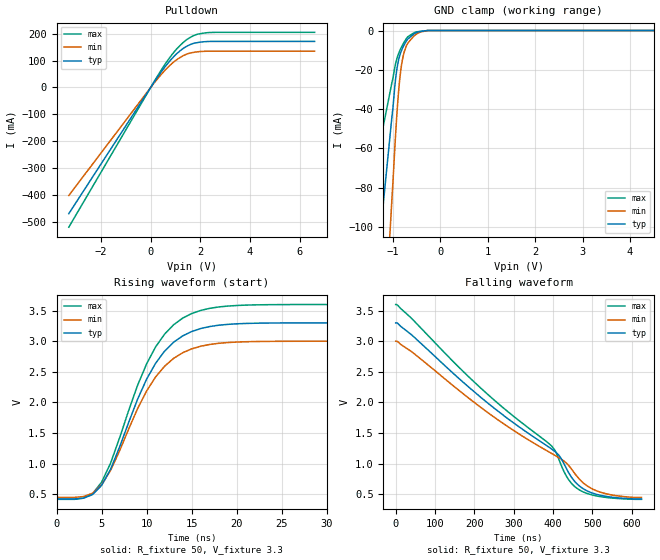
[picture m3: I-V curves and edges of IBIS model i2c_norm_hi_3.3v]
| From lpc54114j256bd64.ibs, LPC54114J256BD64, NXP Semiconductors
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[Model]   i2c_norm_hi_3.3v
Model_type I/O_open_drain
Vinl=8.000E-01
Vinh=2.000E+00
Vref=3.300E+00
Rref=1.000E+03
Cref=0.000E+00
Vmeas=1.650E+00
C_comp   1.270E-12   1.260E-12   1.280E-12
[Voltage Range]   3.300E+00   3.000E+00   3.600E+00
[POWER Clamp Reference]   3.300E+00   3.000E+00   3.600E+00
[GND Clamp Reference]   0.000E+00   0.000E+00   0.000E+00
[Pullup Reference]   3.300E+00   3.000E+00   3.600E+00
[Pulldown Reference]   0.000E+00   0.000E+00   0.000E+00
[Temperature Range]   25   105   -40
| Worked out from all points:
|   slope of the pulldown table from 0 to 0.495 V, typ, clamps not added: 7.43 ohm
|   GND clamp passes 1 mA (typ) near -0.50 V on its own axis
|   rising waveform, R_fixture 50, V_fixture 3.3: 20-80 % time 5.17ns typ, 5.19ns min, 5.15ns max; typ from 0.423 V to 3.3 V
|   falling waveform, R_fixture 50, V_fixture 3.3: 20-80 % time 323ns typ, 336ns min, 314ns max; typ from 3.3 V to 0.423 V
[GND Clamp]
-3.3V     -596.7mA   -1.044A    -303.9mA
-1.02V    -43.83mA   -85.71mA   -26.47mA
-1V       -39.67mA   -77.7mA    -24.42mA
-940mV    -24.04mA   -51.83mA   -16.55mA
-900mV    -17.33mA   -37.22mA   -13.12mA
-860mV    -13.09mA   -25.86mA   -10.57mA
-820mV    -10.26mA   -17.89mA   -8.471mA
-780mV    -8.115mA   -12.67mA   -6.653mA
-720mV    -5.516mA   -8.072mA   -4.267mA
-540mV    -1.504mA   -2.465mA   -1.005mA
-260mV    0A         0A         0A
6.6V      0A         0A         0A
[Pulldown]
-3.3V     -469.8mA   -402.2mA   -520.2mA
340mV     46.54mA    39.26mA    52.17mA
600mV     79.46mA    66.39mA    89.51mA
940mV     115.7mA    95.51mA    131.7mA
1.38V     149.3mA    121.1mA    172.6mA
1.64V     161.2mA    128.8mA    188.4mA
1.86V     166.3mA    132.2mA    197.3mA
2.36V     171mA      134.7mA    204.1mA
6.6V      171.2mA    134.9mA    204.9mA
[Rising Waveform]
R_fixture = 50
V_fixture = 3.3
V_fixture_min = 3.0
V_fixture_max = 3.6
0s        423.3mV    448.4mV    416.8mV
3ns       436.5mV    462.3mV    436mV
5ns       644.7mV    653.1mV    696.5mV
6ns       909.4mV    889.6mV    1.008V
9ns       2.054V     1.9V       2.282V
11ns      2.642V     2.418V     2.909V
13ns      2.984V     2.721V     3.27V
15ns      3.159V     2.875V     3.452V
21ns      3.29V      2.991V     3.59V
46ns      3.3V       3V         3.6V
[Falling Waveform]
R_fixture = 50
V_fixture = 3.3
V_fixture_min = 3.0
V_fixture_max = 3.6
0s        3.3V       3V         3.6V
45ns      3.078V     2.807V     3.343V
216ns     2.085V     1.92V      2.236V
397ns     1.236V     1.165V     1.284V
415ns     1.136V     1.097V     1.069V
434ns     921.1mV    1.01V      796.7mV
458ns     689.6mV    816.5mV    611.2mV
484ns     563.8mV    649.5mV    519.5mV
517ns     487.9mV    541.2mV    464.4mV
625ns     423.3mV    448.4mV    416.8mV
[Ramp]
dV/dt_r   1.7260E+00/5.1170E-09   1.5310E+00/5.1410E-09   1.9099E+00/5.1150E-09
dV/dt_f   1.7260E+00/3.2350E-07   1.5310E+00/3.3613E-07   1.9099E+00/3.1434E-07
R_load = 50
